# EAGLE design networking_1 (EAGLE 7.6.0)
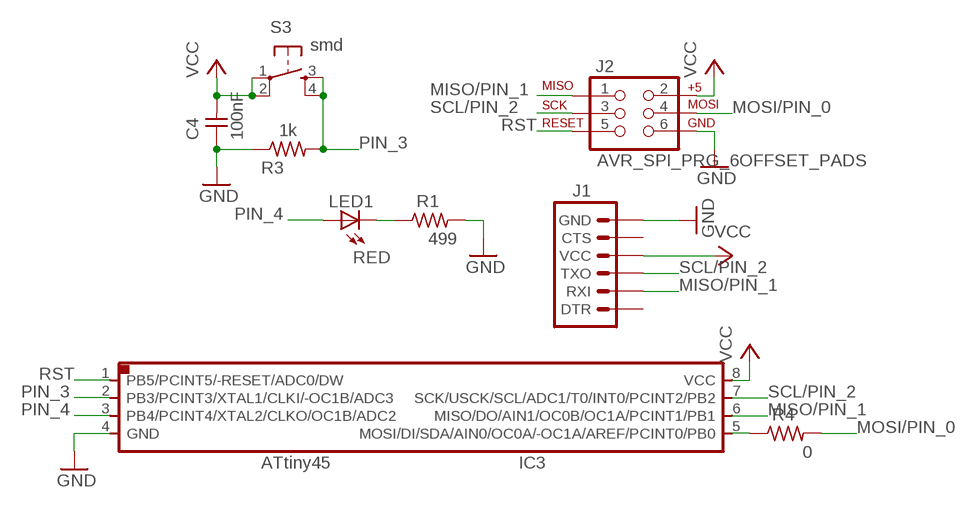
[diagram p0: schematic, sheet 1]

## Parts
C4  100nF  UNPOLARIZED_CAPACITOR1206  [1206]
IC3  ATTINY*5  ATTINY45SI  [SOIC8]
J1  ARDUINO_SERIAL_PROGRAMSMD  [1X06-SMD]
J2  AVR_SPI_PRG_6OFFSET_PADS  [2X3_OFFSET]
LED1  RED  LEDSMT1206  [1206]
R1  499  RESISTOR1206  [1206]
R3  1k  RESISTOR1206  [1206]
R4  0  RESISTOR1206  [1206]
S3  smd  6MM_SWITCH6MM_SWITCH  [6MM_SWITCH]

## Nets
GND: C4.1 IC3.4(GND) J1.6(GND) J2.6 R1.2 R3.1
MISO/PIN_1: IC3.6(MISO/DO/AIN1/OC0B/OC1A/PCINT1/PB1) J1.2(RXI) J2.1
MOSI/PIN_0: J2.4 R4.2
N$1: IC3.5(MOSI/DI/SDA/AIN0/OC0A/-OC1A/AREF/PCINT0/PB0) R4.1
N$3: LED1.C R1.1
PIN_3: IC3.2(PB3/PCINT3/XTAL1/CLKI/-OC1B/ADC3) R3.2 S3.3(S) S3.4(S1)
PIN_4: IC3.3(PB4/PCINT4/XTAL2/CLKO/OC1B/ADC2) LED1.A
RST: IC3.1(PB5/PCINT5/-RESET/ADC0/DW) J2.5
SCL/PIN_2: IC3.7(SCK/USCK/SCL/ADC1/T0/INT0/PCINT2/PB2) J1.3(TXO) J2.3
VCC: C4.2 IC3.8(VCC) J1.4(VCC) J2.2 S3.1(P) S3.2(P1)
Unconnected: J1.1(DTR) J1.5(CTS)

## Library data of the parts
C4 = 01_FAB_Hello:UNPOLARIZED_CAPACITOR: unpolarized_capacitor
IC3 = 01_fab:ATTINY45
J1 = SparkFun-Connectors:ARDUINO_SERIAL_PROGRAM: FTDI connector footprints; PROD_ID: CONN-08971
J2 = SparkFun-Connectors:AVR_SPI_PRG_6: AVR ISP 6 Pin This is the reduced ISP connector for AVR programming. Common on Arduino. This footprint will take up less PCB space and can be used with a 10-pin to 6-pin adapter such as SKU: BOB-08508 **Special note about "TEST_POINT" package. The stop mask is on the top side, so if you want your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
LED1 = led:LED: LED
R1 R3 R4 = 01_FAB_Hello:RESISTOR
S3 = 01_fab:6MM_SWITCH: OMRON SWITCH

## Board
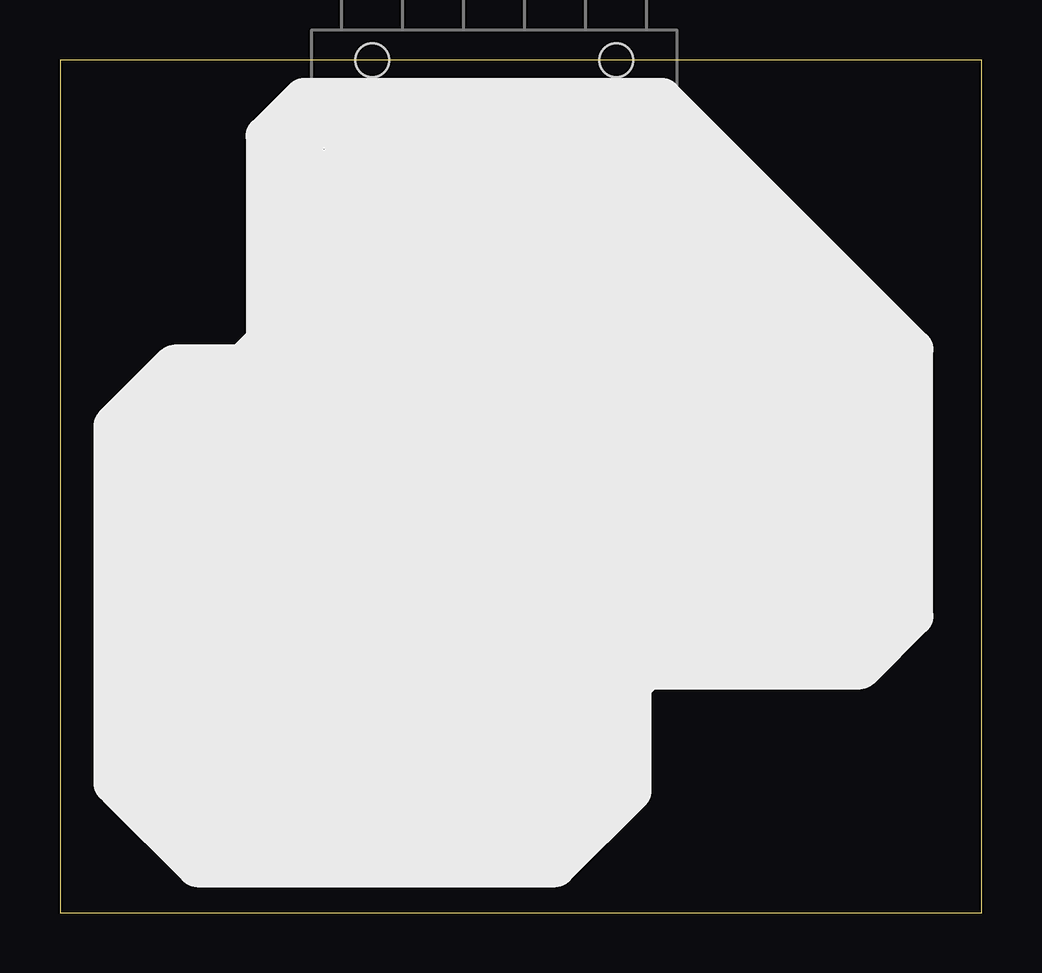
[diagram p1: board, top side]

Size 38.41 x 35.55 mm. Coordinates in mm from the lower left corner, seen from the top.
Outline: 0,0 38.4,0 38.4,35.55 0,35.55 0,0
Copper layers (1*16): Top 0.035mm / dielectric 1.5mm / Bottom 0.035mm
Design rules "default": minimum track width 10mil, minimum drill 24mil, track to track 8mil, track to pad 8mil, pad to pad 8mil, via to via 8mil, smd to smd 8mil, copper to edge 40mil, drill to drill 8mil, minimum pad ring 10mil, minimum via ring 8mil, stop-mask expansion 4mil, vias tented up to drill 0mil, thermal gap 10mil

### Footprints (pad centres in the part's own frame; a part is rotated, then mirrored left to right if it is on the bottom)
1206 = smd 1.6 x 1.803: 1 -1.422,0; 2 1.422,0
SOIC8 = smd 0.5 x 2.2: 1 -1.905,-3.154; 2 -0.645,-3.154; 3 0.625,-3.154; 4 1.895,-3.154; 5 1.905,3.154; 6 0.635,3.154; 7 -0.635,3.154; 8 -1.905,3.154
1X06-SMD = smd 1 x 3: 1 -6.35,5; 2 -3.81,5; 3 -1.27,5; 4 1.27,5; 5 3.81,5; 6 6.35,5 | hole 1.4: -5.08,0; 5.08,0
2X3_OFFSET = drill 1.118 pad 1.88 offset: 1 -2.54,-1.27; 2 -2.54,1.27; 3 0,-1.27; 4 0,1.27; 5 2.54,-1.27; 6 2.54,1.27
1206' = smd 1.6 x 1.803: A -1.422,0; C 1.422,0
6MM_SWITCH = smd 2.286 x 1.524: 1 -3.302,2.286; 2 3.302,2.286; 3 -3.302,-2.286; 4 3.302,-2.286

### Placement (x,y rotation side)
C4  14.61,21.59 90 top
IC3  20,21.59 0 top
J1  18.1,35.56 180 top
J2  30.16,19.05 180 top
LED1  RED  [1206']  12.38,15.24 180 top
R1  6.03,15.24 180 top
R3  8.57,8.89 0 top
R4  30.16,12.7 90 top
S3  20,8.89 270 top

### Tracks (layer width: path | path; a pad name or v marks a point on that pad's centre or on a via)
GND
  Top 0.406: 12.06,20.32 6.67,20.32 4.61,18.26 R1.2 4.61,11.43 R3.1 6.99,8.72 6.99,5.4 8.89,3.49 19.05,3.49 20.32,4.76 20.32,13.97 21.9,15.55 IC3.4 21.9,16.84 23.18,15.56 27.3,15.56 27.62,15.88 J2.6 | 12.06,20.32 14.45,20.32 C4.1 | J1.6 11.75,20.64 12.06,20.32
MISO/PIN_1
  Top 0.406: J2.1 32.7,22.86 30.16,25.4 25.08,25.4 23.81,24.13 23.81,22.86 21.27,22.86 20.64,23.49 IC3.6 20.64,26.99 21.59,27.94 21.59,30.24 J1.2
MOSI/PIN_0
  Top 0.406: R4.2 J2.4
N$1
  Top 0.406: R4.1 30.31,11.43 33.97,11.43 35.24,12.7 35.24,22.86 31.43,26.67 22.54,26.67 21.91,26.03 IC3.5
N$3
  Top 0.406: R1.1 LED1.C
PIN_3
  Top 0.356: IC3.2 19.36,17.13 18.73,16.51 16.19,16.51 14.92,17.78 13.65,17.78 12.38,16.51 12.38,8.89
  Top 0.406: S3.3 17.72,7.62 | 17.72,7.62 S3.4 | R3.2 12.38,8.89 16.45,8.89 17.72,7.62
PIN_4
  Top 0.406: LED1.A 20,15.24 20.63,15.87 IC3.3
RST
  Top 0.406: IC3.1 18.1,19.69 18.73,20.32 J2.5
SCL/PIN_2
  Top 0.406: J1.3 IC3.7 19.37,22.54 20.32,21.59 23.81,21.59 26.35,24.13 29.21,24.13 30.16,23.18 J2.3
VCC
  Top 0.406: J2.2 32.7,13.97 31.43,12.7 23.05,12.7 S3.1 S3.2 22.23,5.53 22.23,4.76 20.32,2.54 5.72,2.54 2.86,5.4 2.86,19.69 5.4,22.23 8.25,22.23 9.53,23.49 9.53,32.07 10.79,33.34 16.19,33.34 16.83,32.7 J1.4 16.83,28.26 18.1,26.99 IC3.8 18.1,23.81 17.3,23.01 C4.2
